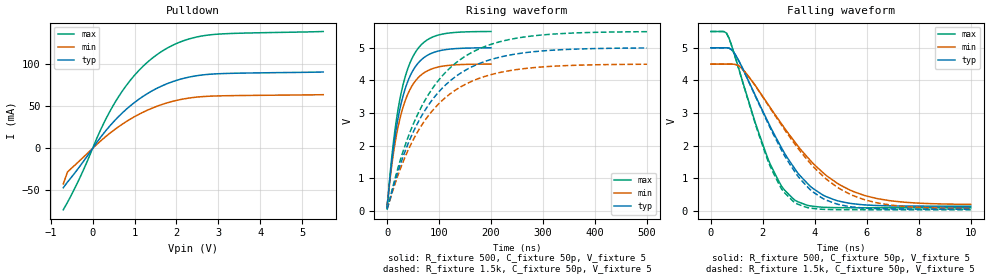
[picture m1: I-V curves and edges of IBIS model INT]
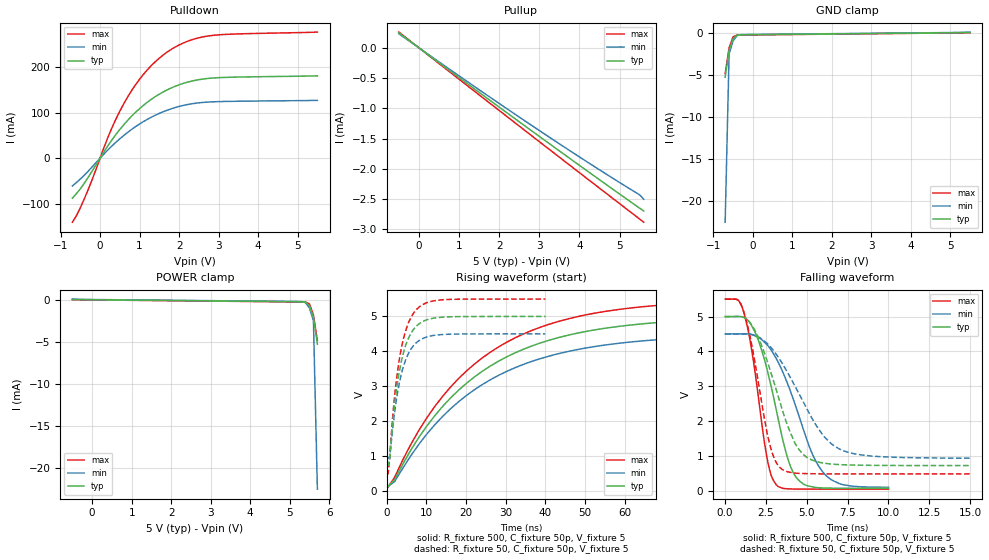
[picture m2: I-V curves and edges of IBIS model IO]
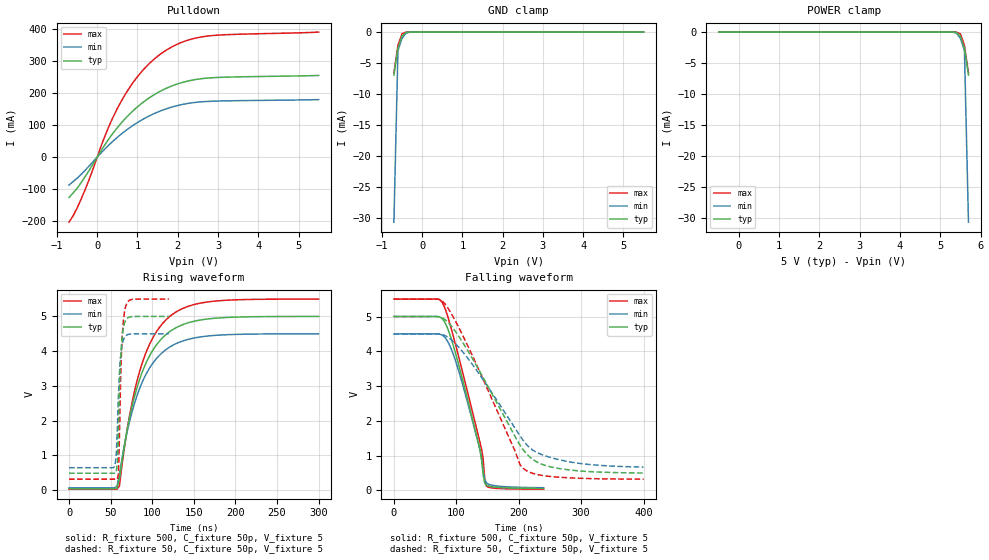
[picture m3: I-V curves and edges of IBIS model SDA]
[IBIS Ver]   3.2
[Comment Char]   |_char
| VDD Nom: 5v, Min: 4.5v, Max: 5.5v
[File name]   pca9674_5v.ibs
[File Rev]   1
[Date]   08-25-2008
[Source]
[Notes]
[Disclaimer]
(C) Copyright 2007 NXP Semiconductors
All rights reserved
NXP Semiconductors (NXP) does not warrant that this model and any other
accompanying information (Model) accurately or fully represents the
operating characteristics and specifications of the semiconductor
products to which the Model relates.  Moreover, the Model is furnished
on an "as is" and with "all faults" basis, and without support or
warranty of any kind.  NXP disclaims all warranties, whether expressed
or implied or statutory, including without limitation all implied
warranties of non-infringement, merchantability and fitness for any
purpose, and those arising from a course of dealing or usage of trade.
NXP does not convey any license under its or any third party's patents,
copyrights or other intellectual property or proprietary rights.
You and your company assume any and all risks and liability arising out
of the application or use of the Model.
In no event shall NXP be liable for any direct, indirect, special,
consequential or incidental damages, however caused, whether in
warranty, contract or tort (including negligence), strict liability or
other legal theory, including, without limitation, for lost profits,
business interruption, or corruption or loss of data or information,
arising out of or in connection with the use of or the inability to use
the Model, even if NXP has been advised of the possibility of such
damages.
NXP provides the Model as a courtesy to our customers. You and your
company shall not distribute, convey, sell, or give the Model to anyone
else without receiving prior written permission from NXP.
NXP reserves the right to make changes without notice to the Model to
improve reliability, function, or design.
Please be aware that your receipt and subsequent use of the Model shall
serve as acceptance of these terms and conditions.  If you do not
accept these terms, return or destroy the Model immediately.
[Copyright]
2008
| SO16 package
[Component]   PCA9674D
Si_location Pin
Timing_location Pin
[Manufacturer]   NXP Semiconductors
[Package]
R_pkg   1.75E-01   1.28E-01   2.11E-01
L_pkg   5.03E-09   3.94E-09   6.26E-09
C_pkg   0.794p   0.715p   0.869p
[Pin] signal_name   model_name   R_pin   L_pin   C_pin
1   AD0   ADDR   1.99E-01  6.26E-09  8.22E-13
2   AD1   ADDR   2.11E-01  5.46E-09  8.69E-13
3   AD2   ADDR   1.56E-01  4.44E-09  7.60E-13
4   P0   IO   1.28E-01  3.94E-09  7.17E-13
5   P1   IO   1.28E-01  3.94E-09  7.15E-13
6   P2   IO   1.56E-01  4.44E-09  7.60E-13
7   P3   IO   2.11E-01  5.46E-09  8.69E-13
8   VSS   GND   1.99E-01  6.26E-09  8.43E-13
9   P4   IO   1.99E-01  6.26E-09  8.43E-13
10   P5   IO   2.11E-01  5.46E-09  8.69E-13
11   P6   IO   1.56E-01  4.44E-09  7.60E-13
12   P7   IO   1.28E-01  3.94E-09  7.17E-13
13   INTb   INT   1.28E-01  3.94E-09  7.15E-13
14   SCL   SCL   1.56E-01  4.44E-09  7.60E-13
15   SDA   SDA   2.11E-01  5.46E-09  8.69E-13
16   VDD   POWER   1.99E-01  6.26E-09  8.43E-13
| TSSOP16 package
[Component]   PCA9674PW
Si_location Pin
Timing_location Pin
[Manufacturer]   NXP Semiconductors
[Package]
R_pkg   3.95E-02   3.52E-02   4.56E-02
L_pkg   1.94n   1.65n   2.40n
C_pkg   .446p   .335p   .771p
[Pin] signal_name   model_name   R_pin   L_pin   C_pin
1   AD0   ADDR   3.52E-02  2.40E-09  4.36E-13
2   AD1   ADDR   3.70E-02  1.93E-09  4.38E-13
3   AD2   ADDR   4.56E-02  1.76E-09  3.45E-13
4   P0   IO   4.00E-02  1.65E-09  3.35E-13
5   P1   IO   4.00E-02  1.65E-09  3.35E-13
6   P2   IO   4.56E-02  1.76E-09  3.45E-13
7   P3   IO   3.70E-02  1.93E-09  4.38E-13
8   VSS   GND   3.52E-02  2.40E-09  4.52E-13
9   P4   IO   3.52E-02  2.40E-09  4.52E-13
10   P5   IO   3.70E-02  1.93E-09  4.38E-13
11   P6   IO   4.56E-02  1.76E-09  3.45E-13
12   P7   IO   4.00E-02  1.65E-09  7.71E-13
13   INTb   ADDR   4.00E-02  1.65E-09  7.71E-13
14   SCL   SCL   4.56E-02  1.76E-09  3.45E-13
15   SDA   SDA   3.70E-02  1.93E-09  4.38E-13
16   VDD   POWER   3.52E-02  2.40E-09  4.52E-13
[Define Package Model]  HVQFN16
[Manufacturer]  ST-NXP Wireless
[OEM]  Unknown
[Description]  Full package model
|[Simulated] Chris Hunat
|[Approved] Wayne Nunn, Roger Real
[Number Of Pins]  16
[Pin Numbers]
|Pin Num   Terminal Name
1   | lead1:pin1
2   | lead2:pin2
3   | lead3:pin3
4   | lead4:pin4
5   | lead5:pin5
6   | lead6:pin6
7   | lead7:pin7
8   | lead8:pin8
9   | lead9:pin9
10   | lead10:pin10
11   | lead11:pin11
12   | lead12:pin12
13   | lead13:pin13
14   | lead14:pin14
15   | lead15:pin15
16   | lead16:pin16
[Model Data]
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[End Model Data]
[End Package Model]
| Models and submodels in the file (5): INT (Open_drain), IO (I/O), SDA (I/O_open_drain), SCL (Input), ADDR (Input)
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[Model]   INT
Model_type Open_drain
Vref=5
Vmeas=2.5
Rref=1.6k
Cref=50p
C_comp   5.2p   5p   5.4p
[Temperature Range] 27   85   -40
[Voltage Range]   5   4.5   5.5
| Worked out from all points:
|   slope of the pulldown table from 0 to 0.75 V, typ, clamps not added: 17 ohm
|   falling waveform, R_fixture 500, C_fixture 50p, V_fixture 5: 20-80 % time 1.97ns typ, 2.6ns min, 1.39ns max; typ from 5 V to 0.139 V
|   falling waveform, R_fixture 1.5k, C_fixture 50p, V_fixture 5: 20-80 % time 1.94ns typ, 2.57ns min, 1.38ns max; typ from 5 V to 0.046 V
|   rising waveform, R_fixture 500, C_fixture 50p, V_fixture 5: 20-80 % time 35.1ns typ, 35.2ns min, 35.1ns max; typ from 0.139 V to 5 V
|   rising waveform, R_fixture 1.5k, C_fixture 50p, V_fixture 5: 20-80 % time 105ns typ, 105ns min, 105ns max; typ from 0.046 V to 4.99 V
[Pulldown]
-700mV    -46.85mA   -42.29mA   -73.04mA
-600mV    -40.09mA   -28.2mA    -64.29mA
-300mV    -21.02mA   -14.28mA   -34.53mA
200mV     13.79mA    9.177mA    23.06mA
400mV     26.03mA    17.52mA    42.92mA
600mV     36.84mA    25.02mA    59.95mA
800mV     46.31mA    31.73mA    74.52mA
1.1V      58.28mA    40.36mA    92.41mA
1.6V      73.01mA    51.21mA    113.7mA
2.1V      82.29mA    58.06mA    126.7mA
2.7V      87.7mA     61.77mA    134.3mA
5.5V      90.74mA    63.79mA    138.9mA
[Falling Waveform]
R_fixture=500
C_fixture=50p
V_fixture=5
V_fixture_min=4.5
V_fixture_max=5.5
0s        5V         4.5V       5.5V
606.1ps   5V         4.5V       5.447V
1.212ns   4.39V      4.353V     3.997V
2.222ns   2.689V     3.242V     1.547V
2.727ns   1.921V     2.659V     744.9mV
3.232ns   1.286V     2.111V     325mV
4.343ns   468.8mV    1.149V     106.1mV
5.556ns   207.4mV    568.6mV    91.02mV
7.071ns   147.1mV    291.7mV    90.25mV
10ns      138.8mV    194.8mV    90.23mV
[Falling Waveform]
R_fixture=1.5k
C_fixture=50p
V_fixture=5
V_fixture_min=4.5
V_fixture_max=5.5
0s        5V         4.5V       5.5V
505.1ps   5V         4.5V       5.498V
707.1ps   4.989V     4.5V       5.285V
1.212ns   4.386V     4.352V     3.984V
2.222ns   2.648V     3.222V     1.478V
2.727ns   1.853V     2.62V      662.2mV
3.232ns   1.195V     2.049V     246.4mV
4.343ns   360.9mV    1.042V     42.71mV
5.556ns   107.5mV    439.9mV    30.39mV
10ns      46.07mV    69.12mV    29.81mV
[Rising Waveform]
R_fixture=500
C_fixture=50p
V_fixture=5
V_fixture_min=4.5
V_fixture_max=5.5
0s        138.7mV    187.4mV    90.23mV
8.081ns   1.37V      1.261V     1.483V
12.12ns   1.904V     1.737V     2.075V
22.22ns   2.921V     2.643V     3.201V
28.28ns   3.363V     3.037V     3.691V
36.36ns   3.81V      3.436V     4.186V
52.53ns   4.372V     3.938V     4.807V
70.71ns   4.694V     4.226V     5.162V
96.97ns   4.891V     4.403V     5.381V
200ns     4.998V     4.498V     5.498V
[Rising Waveform]
R_fixture=1.5k
C_fixture=50p
V_fixture=5
V_fixture_min=4.5
V_fixture_max=5.5
0s        45.97mV    62.61mV    29.81mV
15.15ns   893.7mV    813.7mV    975.5mV
30.3ns    1.633V     1.477V     1.792V
60.61ns   2.739V     2.468V     3.012V
80.81ns   3.267V     2.942V     3.593V
101ns     3.671V     3.305V     4.039V
146.5ns   4.27V      3.842V     4.698V
197ns     4.624V     4.162V     5.088V
262.6ns   4.842V     4.357V     5.327V
500ns     4.993V     4.494V     5.492V
[Ramp]
R_load=1.6k
dV/dt_r   2.974E+0/1.675E-9   2.961E+0/1.840E-9   2.985E+0/1.482E-9
dV/dt_f   2.974E+0/8.642E-11   2.961E+0/1.513E-10   2.985E+0/1.040E-10
|[End   INT
| [End   IO
[Model]   IO
Model_type I/O
Vinh=3.5
Vinl=1.5
Vref=5
Vmeas=2.5
Rref=500
Cref=50p
C_comp   7p   6.8p   7.2p
[Model Spec]
Vinh   1.494   1.195   1.893
Vinl   1.023   0.854   1.563
[Temperature Range] 27   85   -40
[Voltage Range]   5   4.5   5.5
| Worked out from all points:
|   slope of the pulldown table from 0 to 0.75 V, typ, clamps not added: 8.52 ohm
|   slope of the pullup table from 0 to 0.75 V, typ, clamps not added: 2.03 kohm
|   GND clamp passes 1 mA (typ) near -0.52 V on its own axis
|   falling waveform, R_fixture 500, C_fixture 50p, V_fixture 5: 20-80 % time 1.51ns typ, 2.09ns min, 1ns max; typ from 5 V to 0.069 V
|   falling waveform, R_fixture 50, C_fixture 50p, V_fixture 5: 20-80 % time 1.82ns typ, 2.59ns min, 1.16ns max; typ from 5 V to 0.722 V
|   rising waveform, R_fixture 500, C_fixture 50p, V_fixture 5: 20-80 % time 28ns typ, 28.4ns min, 27.6ns max; typ from 0.069 V to 5 V
|   rising waveform, R_fixture 50, C_fixture 50p, V_fixture 5: 20-80 % time 3.48ns typ, 3.5ns min, 3.46ns max; typ from 0.722 V to 5 V
[Pullup]
-500mV    245.4uA    231.5uA    258.8uA
2.5V      -1.222mA   -1.144mA   -1.293mA
4.1V      -1.99mA    -1.846mA   -2.115mA
5.5V      -2.649mA   -2.43mA    -2.829mA
5.6V      -2.696mA   -2.5mA     -2.88mA
[Pulldown]
-700mV    -87.8mA    -60.93mA   -140.7mA
-600mV    -77.8mA    -53.55mA   -126.6mA
-400mV    -54.98mA   -37.53mA   -89.57mA
200mV     27.79mA    18.55mA    46.38mA
400mV     52.28mA    35.22mA    86.09mA
600mV     73.88mA    50.22mA    120.1mA
800mV     92.82mA    63.63mA    149.3mA
1.1V      116.7mA    80.88mA    185mA
1.6V      146.2mA    102.6mA    227.5mA
2.1V      164.7mA    116.2mA    253.5mA
2.7V      175.5mA    123.6mA    268.8mA
5.5V      181.5mA    127.5mA    277.8mA
[GND Clamp]
-700mV    -5.295mA   -22.53mA   -4.852mA
-600mV    -2.115mA   -2.495mA   -1.798mA
-500mV    -736.9uA   -981.7uA   -491.4uA
-400mV    -294uA     -348uA     -283.8uA
-200mV    -239.8uA   -212.7uA   -267.2uA
5.5V      23.22uA    77.99uA    169.3pA
[POWER Clamp]
-500mV    23.22uA    77.99uA    169.3pA
5.2V      -239.8uA   -212.7uA   -267.2uA
5.4V      -294uA     -348uA     -283.8uA
5.5V      -736.9uA   -981.7uA   -491.4uA
5.6V      -2.115mA   -2.495mA   -1.798mA
5.7V      -5.295mA   -22.53mA   -4.852mA
[Falling Waveform]
R_fixture=500
C_fixture=50p
V_fixture=5
V_fixture_min=4.5
V_fixture_max=5.5
0s        5V         4.5V       5.5V
1.111ns   4.983V     4.502V     5.168V
1.616ns   4.743V     4.484V     4.066V
2.626ns   3.367V     4.158V     790.5mV
3.131ns   2.318V     3.793V     169.1mV
3.737ns   1.08V      3.171V     57.77mV
4.242ns   460.2mV    2.53V      47.51mV
5.253ns   120.9mV    1.15V      45.47mV
6.061ns   77.51mV    494.8mV    45.06mV
10ns      69.28mV    98.13mV    44.81mV
[Falling Waveform]
R_fixture=50
C_fixture=50p
V_fixture=5
V_fixture_min=4.5
V_fixture_max=5.5
0s        5V         4.5V       5.5V
1.061ns   4.989V     4.502V     5.254V
1.818ns   4.606V     4.453V     3.701V
2.727ns   3.501V     4.156V     1.328V
3.485ns   2.343V     3.662V     611.1mV
4.242ns   1.394V     3.033V     507.3mV
4.848ns   1.014V     2.492V     493.1mV
6.061ns   792.3mV    1.553V     484.1mV
6.97ns    750.8mV    1.205V     482.4mV
15ns      722.3mV    933.8mV    481.5mV
[Rising Waveform]
R_fixture=500
C_fixture=50p
V_fixture=5
V_fixture_min=4.5
V_fixture_max=5.5
0s        69.03mV    93.83mV    44.8mV
2.02ns    311.4mV    260.4mV    380.9mV
6.061ns   1.155V     994.8mV    1.317V
10.1ns    1.85V      1.62V      2.083V
20.2ns    3.09V      2.74V      3.443V
32.32ns   3.954V     3.528V     4.383V
46.46ns   4.482V     4.014V     4.952V
62.63ns   4.768V     4.28V      5.258V
86.87ns   4.931V     4.433V     5.429V
200ns     5V         4.5V       5.5V
[Rising Waveform]
R_fixture=50
C_fixture=50p
V_fixture=5
V_fixture_min=4.5
V_fixture_max=5.5
0s        722.2mV    930.6mV    481.5mV
404ps     722.2mV    930.6mV    481.8mV
808.1ps   917.4mV    980.2mV    958.8mV
2.02ns    2.46V      2.237V     2.7V
2.828ns   3.158V     2.852V     3.473V
3.636ns   3.663V     3.306V     4.036V
5.253ns   4.304V     3.874V     4.738V
7.677ns   4.738V     4.264V     5.215V
14.14ns   4.981V     4.483V     5.479V
40ns      5V         4.5V       5.5V
[Ramp]
R_load=500
dV/dt_r   6.301E-1/1.024E-9   5.382E-1/1.436E-9   7.243E-1/7.748E-10
dV/dt_f   2.959E+0/3.658E-10   2.644E+0/6.004E-10   3.273E+0/2.083E-10
|[End   IO
| [End   SDA
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[Model]   SDA
Model_type I/O_open_drain
Vinh=3.5
Vinl=1.5
Vref=5
Vmeas=2.5
Rref=1k
Cref=50p
C_comp   6p   5.8p   6.2p
[Model Spec]
[Temperature Range] 27   85   -40
[Voltage Range]   5   4.5   5.5
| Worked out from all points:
|   slope of the pulldown table from 0 to 0.75 V, typ, clamps not added: 5.88 ohm
|   GND clamp passes 1 mA (typ) near -0.52 V on its own axis
|   falling waveform, R_fixture 500, C_fixture 50p, V_fixture 5: 20-80 % time 41.4ns typ, 39.1ns min, 45.5ns max; typ from 5 V to 0.053 V
|   falling waveform, R_fixture 50, C_fixture 50p, V_fixture 5: 20-80 % time 83.3ns typ, 86.1ns min, 78.4ns max; typ from 5 V to 0.498 V
|   rising waveform, R_fixture 500, C_fixture 50p, V_fixture 5: 20-80 % time 35.3ns typ, 35.4ns min, 35.3ns max; typ from 0.047 V to 5 V
|   rising waveform, R_fixture 50, C_fixture 50p, V_fixture 5: 20-80 % time 3.87ns typ, 4.13ns min, 3.67ns max; typ from 0.488 V to 5 V
[Pulldown]
-700mV    -126.5mA   -87.42mA   -203.7mA
-600mV    -112.5mA   -77.06mA   -184.2mA
-400mV    -80.24mA   -54.43mA   -131.7mA
-200mV    -41.6mA    -27.72mA   -69.88mA
200mV     40.47mA    26.71mA    68.47mA
500mV     92.1mA     61.87mA    152mA
700mV     121.1mA    82.16mA    197.1mA
1V        157.3mA    108.2mA    251.7mA
1.5V      201.5mA    140.8mA    315.4mA
2V        229.2mA    161.5mA    353.8mA
2.6V      245.5mA    173.1mA    376.2mA
5.5V      255.4mA    179.8mA    391.2mA
[GND Clamp]
-700mV    -6.935mA   -30.66mA   -6.593mA
-600mV    -2.591mA   -2.99mA    -2.148mA
-500mV    -653.7uA   -1.019mA   -278.6uA
-400mV    -54.45uA   -160.3uA   -7.607uA
-200mV    -25.65nA   -197.3nA   -667.7pA
5.5V      311.2pA    571.6pA    286.3pA
[POWER Clamp]
-500mV    311.2pA    571.6pA    286.3pA
5.2V      -25.65nA   -197.3nA   -667.7pA
5.4V      -54.45uA   -160.3uA   -7.607uA
5.5V      -653.7uA   -1.019mA   -278.6uA
5.6V      -2.591mA   -2.99mA    -2.148mA
5.7V      -6.935mA   -30.66mA   -6.593mA
[Falling Waveform]
R_fixture=500
C_fixture=50p
V_fixture=5
V_fixture_min=4.5
V_fixture_max=5.5
0s        5V         4.5V       5.5V
70.3ns    4.998V     4.499V     5.498V
80ns      4.877V     4.428V     5.315V
101.8ns   3.74V      3.549V     3.978V
135.8ns   1.343V     1.314V     1.536V
140.6ns   855mV      873.4mV    1.176V
143ns     443.6mV    560.4mV    887.1mV
145.5ns   207.4mV    315.8mV    345.9mV
147.9ns   153.8mV    222.2mV    126mV
240ns     53.13mV    74.44mV    33.52mV
[Falling Waveform]
R_fixture=50
C_fixture=50p
V_fixture=5
V_fixture_min=4.5
V_fixture_max=5.5
0s        5V         4.5V       5.5V
68.69ns   4.999V     4.499V     5.5V
80.81ns   4.929V     4.46V      5.384V
96.97ns   4.609V     4.247V     4.921V
121.2ns   3.93V      3.732V     4.047V
202ns     1.3V       1.568V     742.3mV
210.1ns   1.1V       1.366V     590.8mV
230.3ns   805.4mV    1.08V      452.3mV
262.6ns   633.3mV    890.4mV    379.8mV
400ns     498.2mV    668.4mV    321.2mV
[Rising Waveform]
R_fixture=500
C_fixture=50p
V_fixture=5
V_fixture_min=4.5
V_fixture_max=5.5
0s        46.79mV    64.38mV    29.93mV
54.55ns   46.79mV    65.45mV    29.93mV
57.58ns   57.12mV    114mV      29.92mV
60.61ns   321.9mV    447.6mV    122.5mV
72.73ns   2.087V     1.974V     2.147V
84.85ns   3.189V     2.928V     3.418V
103ns     4.114V     3.729V     4.482V
124.2ns   4.615V     4.165V     5.059V
172.7ns   4.943V     4.45V      5.435V
300ns     5V         4.5V       5.5V
[Rising Waveform]
R_fixture=50
C_fixture=50p
V_fixture=5
V_fixture_min=4.5
V_fixture_max=5.5
0s        488mV      647.3mV    317.3mV
53.33ns   488mV      647.7mV    317.3mV
55.76ns   490.7mV    799.3mV    317.3mV
58.18ns   820.9mV    1.85V      324.3mV
59.39ns   1.777V     2.723V     469.6mV
60.61ns   2.939V     3.383V     1.502V
61.82ns   3.71V      3.803V     2.994V
64.24ns   4.503V     4.231V     4.534V
67.88ns   4.882V     4.436V     5.27V
120ns     5V         4.5V       5.5V
[Ramp]
R_load=500
dV/dt_r   2.972E+0/1.196E-9   2.957E+0/1.676E-9   2.984E+0/8.187E-10
dV/dt_f   2.948E+0/4.154E-8   2.907E+0/4.355E-8   2.973E+0/4.126E-8
|[End   SDA
| [End   SCL
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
